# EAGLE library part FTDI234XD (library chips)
FTDI234XD USB to UART Bridge in 3x3 DFN Package
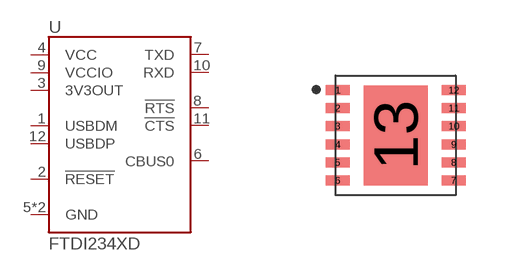
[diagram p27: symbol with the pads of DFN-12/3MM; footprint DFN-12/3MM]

Designator prefix U

## FTDI234XD (DIGIKEY: 768-1178-1-ND; MOUSER: 895-FT234XD-R; NEWARK: 53X3171)  [DFN-12/3MM]
1  USBDM
2  !RESET
3  3V3OUT
4  VCC
5  GND
6  CBUS0
7  TXD
8  !RTS
9  VCCIO
10  RXD
11  !CTS
12  USBDP
13  GND

## Footprint DFN-12/3MM (pad centres in mm)
DFN-12/3MM for FTDI234XD
smd 0.6 x 0.25: 1 -1.45,1.13; 2 -1.45,0.68; 3 -1.45,0.23; 4 -1.45,-0.23; 5 -1.45,-0.68; 6 -1.45,-1.13; 7 1.45,-1.13; 8 1.45,-0.68; 9 1.45,-0.23; 10 1.45,0.23; 11 1.45,0.68; 12 1.45,1.13
smd 1.6 x 2.5: 13 0,0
